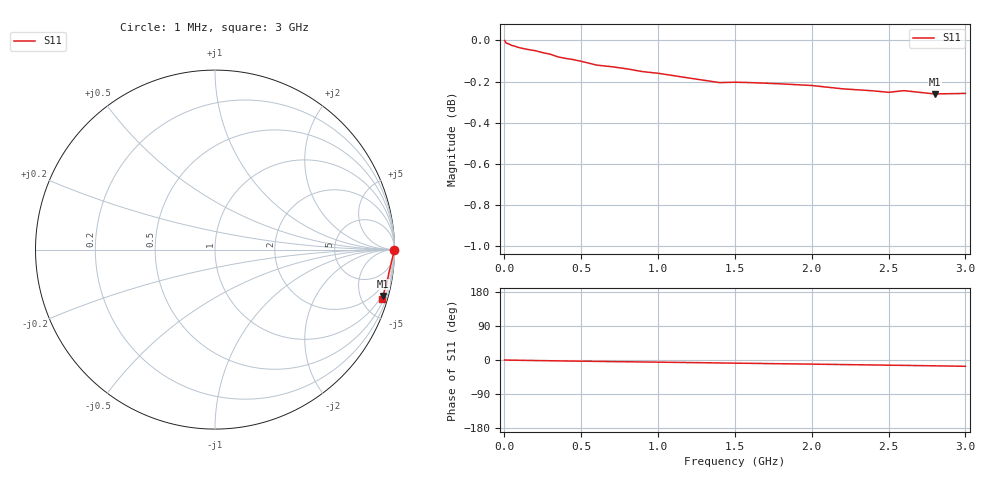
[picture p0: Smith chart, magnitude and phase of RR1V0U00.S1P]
! SIEMENS Small Signal Semiconductors
! BA595
! Si PIN Diode in SOD323
! VR = 1 V
! S-Parameters:  July  1992
# GHz  S  MA  R  50
!  f  S11
! GHz  MAG  ANG
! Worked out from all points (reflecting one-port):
!   33 points, 1 MHz to 3 GHz, reference 50 ohm
!   lowest |S11| = -0.3 dB at 2.8 GHz (marker M1), VSWR 66.80, Z = 41.2 - j365 ohm
!   phase of S11 starts at 0 deg and turns -17 deg over the sweep
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0.001  1 0.0
0.003  0.9998 -0.1
0.01  0.9986 -0.1
0.03  0.998 -0.3
0.05  0.9971 -0.4
0.06  0.997 -0.5
0.08  0.9964 -0.6
0.1  0.9959 -0.8
0.2  0.9943 -1.4
0.35  0.9908 -2.3
0.4  0.99 -2.6
0.45  0.9893 -2.9
0.5  0.9884 -3.1
0.6  0.9863 -3.7
0.8  0.9842 -4.7
0.9  0.9827 -5.2
1  0.9818 -5.7
1.2  0.9792 -6.7
1.4  0.9767 -7.8
1.5  0.9769 -8.3
1.6  0.9767 -8.8
1.8  0.976 -9.9
2  0.9751 -10.9
2.4  0.9722 -13.1
2.5  0.9714 -13.7
2.6  0.9723 -14.2
2.8  0.9705 -15.4
3  0.9708 -16.6
